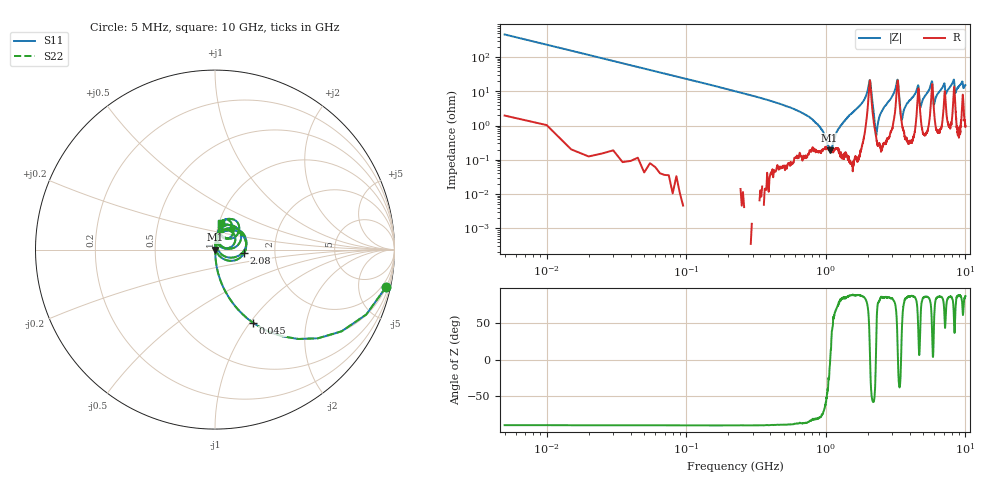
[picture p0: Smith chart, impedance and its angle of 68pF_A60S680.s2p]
! Amotech Co.,Ltd.
! http://www.amotech.co.kr/
! Part Number: A60S680
! These Parameters are Measured in Series Mode Connection
! Operation Temp=25[degC], DC Bias Voltage=0[V]
! Freq. Start=5[MHz] Stop=10[GHz], 2000[Steps]
! Date: Monday, July 13, 2020, 01:43:45
# GHZ S RI R 50.000000
!Freq.(Hz) S11(Real) S11(Imag) S21(Real) S21(Imag) S12(Real) S12(Imag) S22(Real) S22(Imag)
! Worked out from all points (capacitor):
!   2000 points, 5 MHz to 10 GHz, reference 50 ohm
!   read as one part in series: C = 68 pF near 55 MHz
!   lowest |Z| = 187 mohm at 1.065 GHz (marker M1)
!   series resonance near 1.076 GHz, so ESL is about 320 pH
!   S11 on the Smith chart (normalised r, x): 5 MHz: 1.04, -9.20; 45 MHz: 1.00, -1.04; 2.08 GHz: 1.39, -0.06; 10 GHz: 1.02, +0.31
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0.005  0.9541 -0.2072  0.0459 0.2072  0.0459 0.2072  0.9541 -0.2072
0.045  0.2118 -0.4075  0.7882 0.4075  0.7882 0.4075  0.2118 -0.4075
0.155  0.0215 -0.1458  0.9785 0.1458  0.9785 0.1458  0.0215 -0.1458
0.84  0.00209 -0.0124  0.9979 0.0124  0.9979 0.0124  0.00209 -0.0124
1.065  0.00184 -0.000337  0.9982 0.000337  0.9982 0.000337  0.00184 -0.000337
1.31  0.00145 0.0112  0.9986 -0.0112  0.9986 -0.0112  0.00145 0.0112
1.675  0.00219 0.0319  0.9978 -0.0319  0.9978 -0.0319  0.00219 0.0319
2.08  0.1628 -0.0203  0.8372 0.0203  0.8372 0.0203  0.1628 -0.0203
2.3  0.0042 0.00278  0.9958 -0.00278  0.9958 -0.00278  0.0042 0.00278
2.485  0.00227 0.0235  0.9977 -0.0235  0.9977 -0.0235  0.00227 0.0235
3.23  0.1234 0.1147  0.8766 -0.1147  0.8766 -0.1147  0.1234 0.1147
3.34  0.0752 -0.0439  0.9248 0.0439  0.9248 0.0439  0.0752 -0.0439
3.5  0.0118 0.00836  0.9882 -0.00836  0.9882 -0.00836  0.0118 0.00836
4.555  0.0759 0.1066  0.9241 -0.1066  0.9241 -0.1066  0.0759 0.1066
4.75  0.024 0.0222  0.976 -0.0222  0.976 -0.0222  0.024 0.0222
5.005  0.00931 0.0608  0.9907 -0.0608  0.9907 -0.0608  0.00931 0.0608
5.73  0.1119 0.128  0.8881 -0.128  0.8881 -0.128  0.1119 0.128
5.955  0.0281 0.0283  0.9719 -0.0283  0.9719 -0.0283  0.0281 0.0283
6.67  0.0199 0.1069  0.9801 -0.1069  0.9801 -0.1069  0.0199 0.1069
8.335  0.1243 0.0837  0.8757 -0.0837  0.8757 -0.0837  0.1243 0.0837
8.47  0.042 0.0744  0.958 -0.0744  0.958 -0.0744  0.042 0.0744
10  0.0317 0.1476  0.9683 -0.1476  0.9683 -0.1476  0.0317 0.1476
